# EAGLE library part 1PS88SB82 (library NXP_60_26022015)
15 V, 30 mA low Cd Schottky barrier diode Epitaxial low capacitance Schottky barrier diodes encapsulated in very small SMD plastic packages. AAL Eindhoven MK
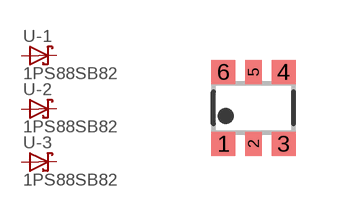
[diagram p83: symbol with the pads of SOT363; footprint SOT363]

Designator prefix -; gates -1=DIODE_SCHOTTKY -2=DIODE_SCHOTTKY -3=DIODE_SCHOTTKY

## 1PS88SB82  [SOT363]
1  -1:A  pas
2  -2:A  pas
3  -3:A  pas
4  -3:K  pas
5  -2:K  pas
6  -1:K  pas

## Footprint SOT363 (pad centres in mm)
SOT363 Plastic surface-mounted package; 6 leads JEDEC: -- IEC: -- JEITA: SC-88
smd 0.6 x 0.6: 1 -0.75,-0.9; 3 0.75,-0.9; 4 0.75,0.9; 6 -0.75,0.9
smd 0.4 x 0.6: 2 0,-0.9; 5 0,0.9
